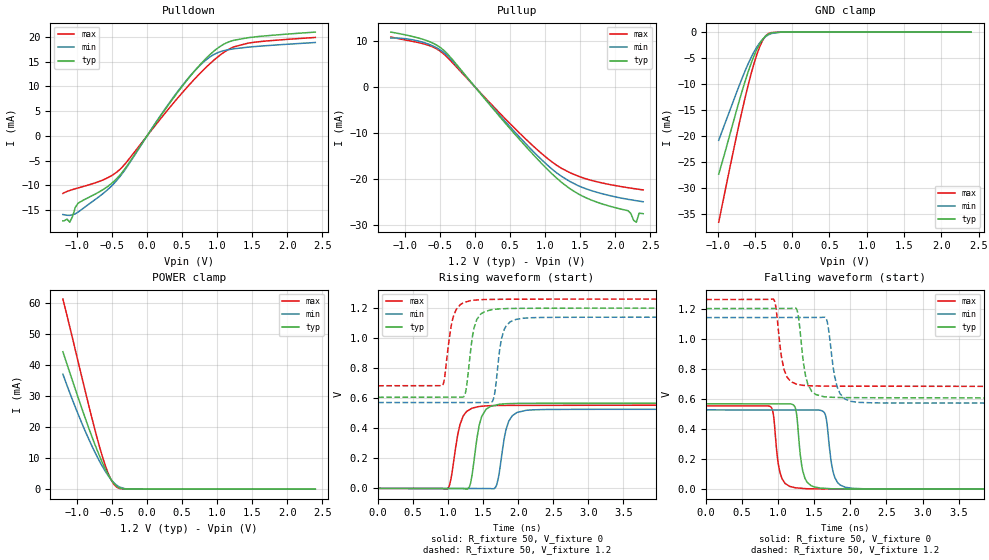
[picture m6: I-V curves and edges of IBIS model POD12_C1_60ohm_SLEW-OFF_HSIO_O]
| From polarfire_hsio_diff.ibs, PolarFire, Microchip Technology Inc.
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|   Model POD12_C1_60ohm_SLEW-OFF_HSIO_O
[Model]   POD12_C1_60ohm_SLEW-OFF_HSIO_O
Model_type   Output
Polarity   Non-Inverting
Enable   Active-High
Vmeas =   0.84
Cref =   5p
Rref =   50
Vref =   0.84
|   typ   min   max
C_comp_pullup   1.335e-12   1.335e-12   1.380e-12
C_comp_pulldown  1.335e-12   1.335e-12   1.380e-12
[Temperature Range]  25C   100C   -40C
[Voltage Range]  1.2   1.14   1.26
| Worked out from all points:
|   slope of the pulldown table from 0 to 0.18 V, typ, clamps not added: 48.1 ohm
|   slope of the pullup table from 0 to 0.18 V, typ, clamps not added: 54.3 ohm
|   GND clamp passes 1 mA (typ) near -0.37 V on its own axis
|   POWER clamp passes 1 mA (typ) near -0.44 V on its own axis
|   rising waveform, R_fixture 50, V_fixture 0: 20-80 % time 115ps typ, 117ps min, 126ps max; typ from 0 V to 0.567 V
|   rising waveform, R_fixture 50, V_fixture 1.2: 20-80 % time 103ps typ, 101ps min, 110ps max; typ from 0.606 V to 1.2 V
|   falling waveform, R_fixture 50, V_fixture 0: 20-80 % time 80ps typ, 86.4ps min, 79.1ps max; typ from 0.567 V to 0 V
|   falling waveform, R_fixture 50, V_fixture 1.2: 20-80 % time 97.5ps typ, 106ps min, 95.4ps max; typ from 1.2 V to 0.606 V
[GND Clamp]
| Voltage   I(typ)   I(min)   I(max)
-984.4mV  -27.36mA   -20.85mA   -36.63mA
-708.7mV  -13.22mA   -10.27mA   -17.58mA
-630mV    -9.442mA   -7.443mA   -12.61mA
-551.3mV  -6.071mA   -4.927mA   -8.091mA
-472.5mV  -3.303mA   -2.86mA    -4.278mA
-433.1mV  -2.213mA   -2.035mA   -2.745mA
-393.7mV  -1.354mA   -1.365mA   -1.538mA
-354.4mV  -738.1uA   -853.7uA   -711.7uA
-315mV    -352.4uA   -492.8uA   -262uA
-157.5mV  -6.952uA   -25.53uA   -1.531uA
-39.38mV  -223.3nA   -1.393uA   -60.97nA
2.4V      0A         0A         0A
[POWER Clamp]
| Voltage   I(typ)   I(min)   I(max)
-1.2V     44.33mA    37.08mA    61.33mA
-1.063V   34.96mA    28.78mA    48.72mA
-905.6mV  24.47mA    19.99mA    33.89mA
-787.5mV  17.03mA    14mA       23.06mA
-669.4mV  10.26mA    8.667mA    13.03mA
-590.6mV  6.299mA    5.605mA    7.313mA
-551.3mV  4.569mA    4.255mA    4.935mA
-472.5mV  1.839mA    2.031mA    1.558mA
-433.1mV  941.2uA    1.284mA    654.9uA
-315mV    34.81uA    149.8uA    11.13uA
-236.2mV  2.462uA    44.69uA    773.7nA
2.4V      0A         0A         0A
[Pullup]
| Voltage   I(typ)   I(min)   I(max)
-1.2V     11.9mA     10.61mA    10.83mA
-748.1mV  10.36mA    9.712mA    9.406mA
-433.1mV  7.788mA    7.317mA    6.984mA
675mV     -12.08mA   -11.54mA   -10.61mA
1.239V    -20.78mA   -19.46mA   -17.73mA
1.633V    -24.41mA   -22.39mA   -20.18mA
2.184V    -26.9mA    -24.42mA   -21.9mA
2.224V    -27.5mA    -24.52mA   -21.99mA
2.263V    -28.97mA   -24.62mA   -22.08mA
2.303V    -29.38mA   -24.71mA   -22.17mA
2.342V    -27.42mA   -24.81mA   -22.25mA
2.4V      -27.54mA   -24.95mA   -22.37mA
[Pulldown]
| Voltage   I(typ)   I(min)   I(max)
-1.2V     -17.14mA   -15.85mA   -11.6mA
-1.142V   -16.78mA   -16.01mA   -11.21mA
-1.103V   -17.4mA    -16.02mA   -11mA
-984.4mV  -13.58mA   -15.38mA   -10.5mA
-590.6mV  -10.49mA   -11.2mA    -8.643mA
-393.7mV  -8.027mA   -8.333mA   -6.847mA
412.5mV   8.335mA    8.498mA    7.225mA
675mV     13.04mA    13.05mA    11.42mA
900mV     16.43mA    15.95mA    14.6mA
1.125V    18.71mA    17.29mA    17.12mA
1.436V    19.8mA     17.89mA    18.69mA
2.4V      20.94mA    18.84mA    19.86mA
[Ramp]
dV/dt_r   0.340476/0.114691n  0.316039/0.117198n  0.332061/0.126156n
dV/dt_f   0.356127/97.4762p  0.341012/0.106137n  0.34613/95.3902p
R_load = 50
[Rising Waveform]
R_fixture = 50
V_fixture = 0
V_fixture_min = 0
V_fixture_max = 0
| Time   V(typ)   V(min)   V(max)
0s        1.174uV    1.428uV    1.75uV
987ps     -686.7uV   -482.7uV   -4.068mV
1.167ns   -812.2uV   -571uV     424.8mV
1.301ns   9.613mV    -636.7uV   523.2mV
1.434ns   400.5mV    -701.9uV   544.5mV
1.54ns    527.3mV    -753.9uV   548.9mV
1.679ns   554.3mV    10.73mV    551.3mV
1.862ns   564mV      446.1mV    552.4mV
2.117ns   566.2mV    520.3mV    552.6mV
10ns      567.5mV    526.7mV    553.4mV
[Rising Waveform]
R_fixture = 50
V_fixture = 1.2
V_fixture_min = 1.14
V_fixture_max = 1.26
| Time   V(typ)   V(min)   V(max)
0s        606.4mV    571.6mV    683.1mV
913ps     607mV      571.6mV    685.1mV
1.058ns   607.1mV    571.6mV    1.118V
1.221ns   610.2mV    571.6mV    1.236V
1.264ns   688.3mV    571.6mV    1.242V
1.369ns   1.07V      571.6mV    1.253V
1.631ns   1.19V      580.1mV    1.258V
1.799ns   1.196V     1.058V     1.259V
2.07ns    1.198V     1.132V     1.259V
10ns      1.2V       1.14V      1.26V
[Falling Waveform]
R_fixture = 50
V_fixture = 0
V_fixture_min = 0
V_fixture_max = 0
| Time   V(typ)   V(min)   V(max)
0s        567.5mV    526.7mV    553.4mV
896ps     566.9mV    526.2mV    546.6mV
1.022ns   566.8mV    526.2mV    113.8mV
1.237ns   537.9mV    526mV      9.356mV
1.37ns    71.99mV    526mV      3.826mV
1.583ns   7.414mV    523.9mV    1.52mV
1.663ns   5.014mV    474.3mV    1.317mV
1.785ns   2.178mV    76.09mV    1.008mV
2.028ns   1.167mV    5.723mV    659.2uV
10ns      2.416uV    3.544uV    2.611uV
[Falling Waveform]
R_fixture = 50
V_fixture = 1.2
V_fixture_min = 1.14
V_fixture_max = 1.26
| Time   V(typ)   V(min)   V(max)
0s        1.2V       1.14V      1.26V
938ps     1.201V     1.141V     1.26V
1.08ns    1.201V     1.141V     794.3mV
1.26ns    1.19V      1.141V     696.1mV
1.341ns   871.1mV    1.141V     690mV
1.464ns   648.8mV    1.141V     686.6mV
1.665ns   612.8mV    1.133V     685.1mV
1.816ns   609.4mV    679.7mV    684.6mV
2.015ns   608.1mV    582.7mV    684.2mV
10ns      606.4mV    571.6mV    683.1mV
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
